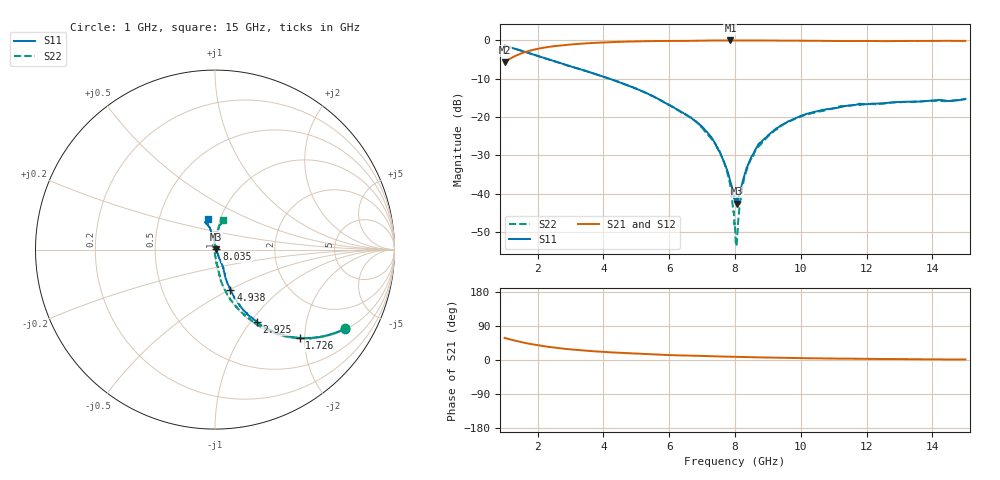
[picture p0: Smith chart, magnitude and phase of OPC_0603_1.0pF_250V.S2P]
! FILE NAME
! DATE 08/21/2012  11:59
! CORRECTED  DATA
# GHz  S  MA  R  50.00
!  FREQ  S11M  S11A  S21M  S21A  S12M  S12A  S22M  S22A
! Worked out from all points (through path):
!   1601 points, 1 GHz to 15 GHz, reference 50 ohm
!   highest |S21| = -0.07 dB at 7.86 GHz (marker M1); lowest = -5.7 dB at 1 GHz (marker M2)
!   lowest |S11| = -42.6 dB at 8.053 GHz (marker M3), VSWR 1.01, Z = 50.7 + j0.248 ohm
!   |S11| at or under -10 dB: 4.175 GHz to end of sweep
!   |S22| runs from -53.6 to -1.4 dB; largest |S21 - S12| = 0.0082
!   S11 on the Smith chart (normalised r, x): 1 GHz: 1.04, -3.27; 1.726 GHz: 1.03, -1.89; 2.925 GHz: 1.04, -1.08; 4.938 GHz: 1.07, -0.50; 8.035 GHz: 1.02, +0.00; 15 GHz: 0.88, +0.30
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1  0.8488 -31.2  0.5162 58.4  0.5162 58.3  0.8489 -31.2
1.72625  0.682 -46.2  0.7213 43.3  0.7209 43.4  0.6822 -46.4
2.925  0.4659 -59.9  0.8737 28.6  0.8732 28.7  0.4676 -61.4
3.33625  0.414 -62.8  0.9009 25.6  0.9006 25.6  0.4129 -64.8
4.9375  0.2393 -68.9  0.9622 16.9  0.9615 16.9  0.2397 -75.8
5.6725  0.1713 -69.7  0.976 14.1  0.9758 14.1  0.1706 -79.6
6.7225  0.09315 -65.0  0.9819 11.4  0.9819 11.4  0.09296 -81.5
7.29125  0.05394 -63.9  0.9886 10.0  0.9887 10.0  0.05162 -84.9
7.615  0.02936 -56.3  0.99 9.2  0.9902 9.2  0.02949 -89.3
7.78125  0.01933 -47.4  0.9908 8.9  0.9905 8.9  0.01761 -94.1
7.86  0.01437 -38.9  0.9914 8.7  0.9908 8.7  0.01264 -97.9
8  0.008507 -1.7  0.9911 8.4  0.9904 8.4  0.003775 -128.2
8.035  0.007754 9.9  0.9912 8.3  0.9904 8.3  0.002096 -166.4
8.0525  0.007436 19.2  0.9912 8.3  0.9914 8.2  0.002228 162.9
8.0875  0.007911 40.3  0.9909 8.2  0.991 8.2  0.003814 131.4
8.1925  0.01224 69.2  0.9903 8.0  0.9904 8.0  0.00963 101.4
8.28875  0.0176 81.8  0.9901 7.8  0.9903 7.8  0.01663 96.1
8.6475  0.03943 95.5  0.9891 7.2  0.9892 7.2  0.03847 89.0
9.40875  0.07824 100.5  0.9875 5.9  0.9871 5.9  0.07664 86.3
10.33625  0.1144 102.5  0.9824 4.5  0.9821 4.5  0.112 80.7
12.6725  0.1534 108.9  0.9711 2.7  0.971 2.7  0.1517 76.3
15  0.1724 102.7  0.9795 1.6  0.979 1.6  0.1713 75.1
